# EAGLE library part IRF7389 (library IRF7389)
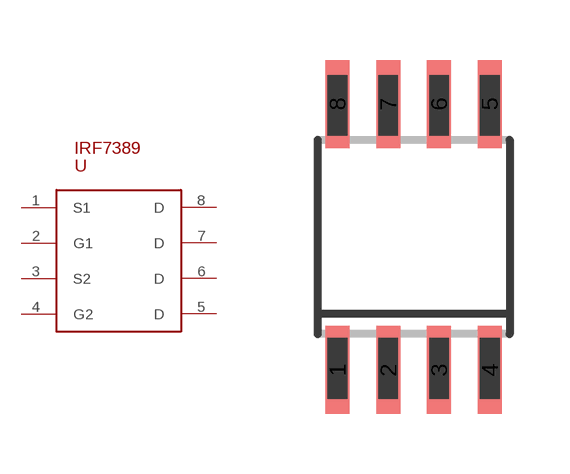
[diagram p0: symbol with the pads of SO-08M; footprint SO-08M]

Designator prefix U

## IRF7389  [SO-08M]
1  S1
2  G1
3  S2
4  G2
5  D
6  D
7  D
8  D

## Footprint SO-08M (pad centres in mm)
Small Outline Medium Plastic Gull Wing 207-mil body, package type SM
smd 0.6 x 2.2: 1 -1.905,-3.33; 2 -0.635,-3.33; 3 0.635,-3.33; 4 1.905,-3.33; 5 1.905,3.33; 6 0.635,3.33; 7 -0.635,3.33; 8 -1.905,3.33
